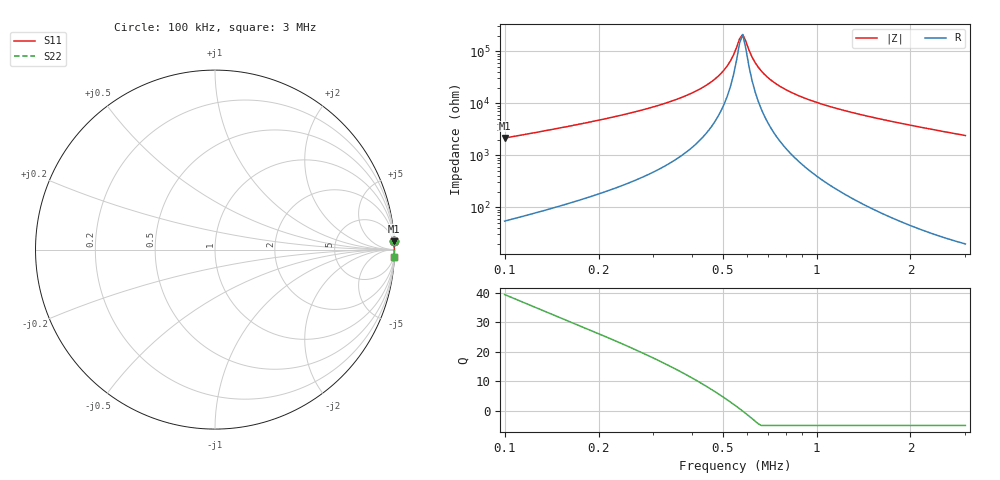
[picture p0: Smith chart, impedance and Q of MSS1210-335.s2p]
# MHz S MA R 50
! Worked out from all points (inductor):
!   150 points, 100 kHz to 3 MHz, reference 50 ohm
!   read as one part in series: L = 3.29 mH near 100 kHz
!   highest Q = 39.4 at 100 kHz (marker M1), where L = 3.4 mH
!   self-resonance near 566.8 kHz
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0.1  0.9977 2.7  0.04669 -85.9  0.04669 -85.9  0.9977 2.7
0.1769453  0.9988 1.4  0.02469 -86.6  0.02469 -86.6  0.9988 1.4
0.3673442  0.9994 0.4  0.007839 -85.2  0.007839 -85.2  0.9994 0.4
0.4409423  0.9994 0.3  0.004595 -83.0  0.004595 -83.0  0.9994 0.3
0.4830989  0.9995 0.2  0.003045 -80.1  0.003045 -80.1  0.9995 0.2
0.5173408  0.9995 0.1  0.001912 -74.8  0.001912 -74.8  0.9995 0.1
0.5415067  0.9995 0.1  0.001186 -65.6  0.001186 -65.6  0.9995 0.1
0.5668015  0.9995 0.0  0.0005741 -33.7  0.0005741 -33.7  0.9995 0.0
0.5798886  0.9995 -0.0  0.0004765 7.5  0.0004765 7.5  0.9995 -0.0
0.5932778  0.9995 -0.0  0.0006442 43.5  0.0006442 43.5  0.9995 -0.0
0.6209909  0.9995 -0.1  0.00129 69.2  0.00129 69.2  0.9995 -0.1
0.6499985  0.9996 -0.1  0.002022 77.1  0.002022 77.1  0.9996 -0.1
0.6803611  0.9996 -0.2  0.002776 80.8  0.002776 80.8  0.9996 -0.2
0.7285849  0.9996 -0.2  0.00393 83.6  0.00393 83.6  0.9996 -0.2
0.7982418  0.9996 -0.3  0.005506 85.4  0.005506 85.4  0.9996 -0.3
0.8745582  0.9996 -0.4  0.007131 86.4  0.007131 86.4  0.9996 -0.4
1.074016  0.9996 -0.6  0.01103 87.5  0.01103 87.5  0.9996 -0.6
1.289197  0.9996 -0.9  0.01489 87.8  0.01489 87.8  0.9996 -0.9
1.583221  0.9995 -1.1  0.01982 87.9  0.01982 87.9  0.9995 -1.1
2.035123  0.9993 -1.5  0.02702 87.8  0.02702 87.8  0.9993 -1.5
2.556974  0.9991 -2.0  0.03503 87.5  0.03503 87.5  0.9991 -2.0
3  0.9988 -2.4  0.0417 87.1  0.0417 87.1  0.9988 -2.4
